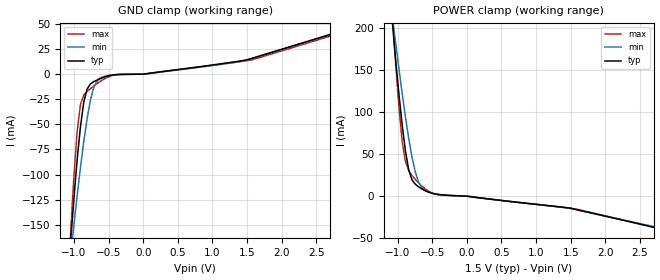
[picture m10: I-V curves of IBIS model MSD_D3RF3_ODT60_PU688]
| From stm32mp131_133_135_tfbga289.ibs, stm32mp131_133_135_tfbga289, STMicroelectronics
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[Model] MSD_D3RF3_ODT60_PU688
Model_type   Input
C_comp 2.378pF   2.331pF   2.439pF
Vinh = 925.000mV
Vinl = 575.000mV
[Temperature Range]   25.000   125.000   -40.000
[Voltage Range]   1.500V   1.425V   1.575V
[GND Clamp Reference]   0.00V   0.00V   0.00V
[POWER Clamp Reference]   1.500V   1.425V   1.575V
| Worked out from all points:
|   GND clamp passes 1 mA (typ) near -0.45 V on its own axis
|   POWER clamp passes 1 mA (typ) near -0.27 V on its own axis
[GND Clamp]
-1.48V    -604.4mA   -472.3mA   -811.3mA
-1.05V    -167.4mA   -181.1mA   -159.3mA
-1.002V   -124.5mA   -150.7mA   -102.4mA
-954.6mV  -85.47mA   -121.1mA   -57.15mA
-906.8mV  -52.42mA   -93.18mA   -30.13mA
-859.1mV  -28mA      -67.27mA   -20.87mA
-811.4mV  -14.82mA   -44.5mA    -17.25mA
-715.9mV  -7.509mA   -13.51mA   -11.83mA
-668.2mV  -5.851mA   -6.749mA   -9.37mA
-525mV    -2.105mA   -1.626mA   -3.31mA
1.48V     14.06mA    13.9mA     13.34mA
2.959V    45.15mA    44.47mA    43.33mA
[Power Clamp]
-1.459V   601.9mA    477.9mA    800.7mA
-1.077V   208.5mA    214.9mA    220.5mA
-1.03V    163.7mA    183.3mA    160.2mA
-981.8mV  122.3mA    152.4mA    106.8mA
-934.1mV  84.97mA    122.6mA    65.26mA
-886.4mV  53.61mA    94.29mA    40.88mA
-838.6mV  31.01mA    68.43mA    30.33mA
-790.9mV  19.26mA    46.03mA    24.55mA
-695.5mV  11.01mA    16.4mA     15.61mA
-456.8mV  2.534mA    2.761mA    2.535mA
1.5V      -14.3mA    -14.78mA   -14.49mA
2.98V     -42.24mA   -41mA      -42.32mA
